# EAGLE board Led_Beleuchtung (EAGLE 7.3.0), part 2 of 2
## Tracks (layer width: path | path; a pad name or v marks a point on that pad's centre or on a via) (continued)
N$54  (via drill 0.35 pad 0.7) (continued)
  Bottom 0.7: v74.39,103.48 v75.04,102.83 v75.19,103.68 v74.54,104.33 v73.74,104.13 v74.39,103.48 | v74.39,103.48 74.64,103.73 | v64.14,114.98 v64.79,114.33 v64.94,115.18 v64.29,115.83 v63.49,115.63 v64.14,114.98 | v64.14,114.98 64.39,115.23
  Bottom 1.2: 74.64,103.73 74.64,105.03 64.44,115.23 64.39,115.23
N$55  (via drill 0.35 pad 0.7)
  Top 0.3: 70.54,99.66 v70.54,99.18 | 51.31,103.57 v50.96,103.57
  Top 0.7: v50.96,103.57 v50.96,102.65 v51.67,103.15 v51.67,104.06 v50.96,104.49 v50.96,103.57 | v50.96,103.57 51.32,103.57 | v69.69,99.33 v69.04,98.68 v69.89,98.53 v70.54,99.18 v70.34,99.98 v69.69,99.33 | v69.69,99.33 69.94,99.08
  Top 0.8: 71.54,100.64 D53.C
  Top 1.2: D53.C 70.54,99.66 | D54.A 51.31,103.57
  Bottom 0.3: 51.31,103.57 v50.96,103.57 | 70.08,99.18 v70.54,99.18
  Bottom 0.7: v50.96,103.57 v50.96,102.65 v51.67,103.15 v51.67,104.06 v50.96,104.49 v50.96,103.57 | v50.96,103.57 51.32,103.57 | v69.69,99.33 v69.04,98.68 v69.89,98.53 v70.54,99.18 v70.34,99.98 v69.69,99.33 | v69.69,99.33 69.94,99.08
  Bottom 1.2: 51.31,103.57 51.31,96.58 53.11,94.78 arc-33 62,93.25 64.87,93.97 70.08,99.18
N$56
  Top 0.7: IC16.3 53.94,119.88
  Top 0.8: 57.13,120.15 C67.2 56.53,120.33 53.94,119.88 | 57.87,117.15 R43.1
  Top 1.2: R43.1 57.13,120.15 | D54.C 51.31,110.76 52.57,112.02 54.36,112.02 57.87,115.52 57.87,117.15
N$57
  Top 0.5: IC17.1 15.22,88.5
  Top 0.8: 15.22,88.5 14.82,85.92 C69.1
  Top 1.2: C69.1 14.65,84.65 15.4,83.61 D56.C
N$58
  Top 1.2: D55.1 19.45,83.44 18.92,83.05 D56.A
N$59
  Top 0.78: IC17.6 12.08,89.18
  Top 0.8: 12.08,89.18 11.31,88.63 D57.C | 12.8,78.53 L27.1
  Top 1.2: D57.C C69.2 12.31,82.67 13.25,81.38 12.8,78.53
N$60
  Top 0.8: 4.22,87.05 C70.2 | 4.77,79.8 L27.2
  Top 1.2: 4.77,79.8 5.2,82.53 3.81,84.44 4.22,87.05 3.12,87.23 2.59,87.96 3.25,92.09 7.75,95.37 C71.1 16.14,97.34 16.61,97.81 16.79,97.98 30.69,97.98 D58.A
N$61
  Bottom 0.5: D6.A 27.63,15.54 R5.1
N$62  (via drill 0.35 pad 0.7)
  Top 0.6: IC17.3 15.59,90.73
  Top 0.7: v22.43,90.66 v22.43,91.58 v21.73,91.09 v21.73,90.17 v22.43,89.74 v22.43,90.66 | v22.43,90.66 22.08,90.66 | v23.35,74.29 v22.65,74.71 v22.65,75.63 v23.35,76.13 | v23.35,75.21 v23.35,76.13 | v23.35,74.29 v23.35,75.21 | v23.35,75.21 23,75.21 | 22.14,91.33 22.14,90.96 v22.43,90.66 | v23.35,76.13 24,76.13 24.09,76.03 | v23.35,74.29 24.19,74.28
  Top 0.8: 16.33,93.92 C71.2 16.04,93.48 15.59,90.73
  Top 1.2: 16.33,93.92 R45.1 19.93,93.49 22.14,91.33 | D59.C 24.54,75.21 v23.35,75.21
  Bottom 0.7: v22.43,90.66 v22.43,91.58 v21.73,91.09 v21.73,90.17 v22.43,89.74 v22.43,90.66 | v22.43,90.66 22.08,90.66 | v23.35,75.21 v23.35,76.13 v22.65,75.63 v22.65,74.71 v23.35,74.29 v23.35,75.21 | v23.35,75.21 23,75.21
  Bottom 1.2: 23,75.21 22.09,76.11 22.09,90.65 22.08,90.66
N$63
  Top 0.5: IC10.1 81.45,47.83
  Top 0.8: 81.45,47.83 83.29,49.66 C41.1
  Top 1.2: C41.1 84.17,50.59 84.17,51.87 D21.C
N$64
  Top 1.2: D20.1 81,54.39 81.66,54.39 D21.A
N$65
  Top 0.78: IC10.6 83.58,45.44
  Top 0.8: 83.58,45.44 84.71,45.41 86.06,46.76 D22.C | 89.27,54.45 L20.1
  Top 1.2: D22.C C41.2 87.14,50.73 87.14,52.32 89.27,54.45
N$66  (via drill 0.35 pad 0.7)
  Top 0.7: v70.54,45.99 v69.62,45.99 v70.12,45.28 v71.04,45.28 v71.46,45.99 v70.54,45.99 | v70.54,45.99 70.54,45.63 | v52.24,46.85 v51.81,46.14 v50.89,46.14 v50.4,46.85 | v51.32,46.85 v50.4,46.85 | v52.24,46.85 v51.32,46.85 | v51.32,46.85 51.32,46.49 | v50.4,46.85 50.4,47.78 50.59,47.78 | v52.24,46.85 52.24,47.73 51.84,47.73
  Top 0.8: 91.2,42.52 C42.2 | 95.04,48.71 L20.2
  Top 1.2: 95.04,48.71 92.98,46.65 92.98,44.3 91.2,42.52 91.99,41.73 91.99,40.83 89.02,37.87 83.46,37.87 C43.1 75.16,41.83 71.36,45.63 70.54,45.63 | D23.A 51.31,46.85 v51.32,46.85
  Bottom 0.7: v70.54,45.99 v69.62,45.99 v70.12,45.28 v71.04,45.28 v71.46,45.99 v70.54,45.99 | v70.54,45.99 70.54,45.63 | v51.32,46.85 v50.4,46.85 v50.89,46.14 v51.81,46.14 v52.24,46.85 v51.32,46.85 | v51.32,46.85 51.32,46.49
  Bottom 1.2: 51.32,46.49 52.23,45.58 70.49,45.58 70.54,45.63
N$67  (via drill 0.35 pad 0.7)
  Top 0.3: 51.31,54.86 v51.67,54.86
  Top 0.7: v69.34,58.83 v69.99,58.18 v70.14,59.03 v69.49,59.68 v68.69,59.48 v69.34,58.83 | v69.34,58.83 69.59,59.08 | v50.96,54.37 v50.96,53.45 v51.67,53.95 v51.67,54.86 v50.96,55.29 v50.96,54.37 | v50.96,54.37 51.32,54.37
  Top 0.8: D23.C
  Top 1.2: 69.59,59.08 D24.A | D23.C 51.31,54.86
  Route3 0.3: 51.3,54.37 v50.96,54.37
  Route3 0.7: v69.34,58.83 v69.99,58.18 v70.14,59.03 v69.49,59.68 v68.69,59.48 v69.34,58.83 | v69.34,58.83 69.59,59.08 | v50.96,54.37 v50.96,53.45 v51.67,53.95 v51.67,54.86 v50.96,55.29 v50.96,54.37 | v50.96,54.37 51.32,54.37
  Route3 1.2: 69.59,59.08 66.31,62.36 63.61,63.08 arc-35 53.11,61.01 51.3,59.21 51.3,54.37
N$68
  Top 0.7: IC10.3 79.84,46.23
  Top 0.8: 77.37,44.08 C43.2 77.99,44.28 79.84,46.23 | 75.43,46.05 R31.1
  Top 1.2: R31.1 77.37,44.08 | D24.C 75.47,53.2 75.47,51.76 73.4,49.7 73.4,48.08 75.43,46.05
N$69
  Top 0.8: 26.42,108.22 C45.1 26.42,108.22 | IC11.1 26.42,108.22
  Top 1.2: C45.1 25.54,107.28 25.54,106 D26.C
N$70
  Top 1.2: D25.1 28.71,103.49 28.05,103.49 D26.A
N$71
  Top 0.78: IC11.6 26.31,112.33
  Top 0.8: D27.C 25.04,112.33 26.31,112.33 | 20.44,103.43 L21.1
  Top 1.2: D27.C C45.2 22.66,107.24 22.66,105.65 20.44,103.43
N$72  (via drill 0.35 pad 0.7)
  Top 0.7: v57.7,110.89 v58.12,111.59 v59.04,111.59 v59.54,110.89 | v58.62,110.89 v59.54,110.89 | v57.7,110.89 v58.62,110.89 | v58.62,110.89 58.62,111.24 | v40.99,111.82 v41.91,111.82 v41.42,112.52 v40.5,112.52 v40.07,111.82 v40.99,111.82 | v40.99,111.82 40.99,112.17 | v57.7,110.89 57.7,110.03 57.69,110.03 | v59.54,110.89 59.54,109.78 59.39,109.78
  Top 0.8: 18.52,115.36 C46.2 | 14.7,109.17 L21.2
  Top 1.2: 18.52,115.36 17.72,116.15 17.72,117.05 20.69,120.01 26.26,120.01 C47.1 34,116.05 37.87,112.17 40.99,112.17 | C46.2 16.74,113.55 16.74,111.21 14.7,109.17 | D28.A 58.67,110.89 v58.62,110.89
  Bottom 0.7: v58.62,110.89 v59.54,110.89 v59.04,111.59 v58.12,111.59 v57.7,110.89 v58.62,110.89 | v58.62,110.89 58.62,111.24 | v40.99,111.82 v41.91,111.82 v41.42,112.52 v40.5,112.52 v40.07,111.82 v40.99,111.82 | v40.99,111.82 40.99,112.17
  Bottom 1.2: 58.62,111.24 57.67,112.18 41.01,112.18 40.99,112.17
N$73  (via drill 0.35 pad 0.7)
  Top 0.3: 40.16,98.93 v40.64,98.93 | 58.67,103.4 v59.02,103.4
  Top 0.7: v59.02,103.4 v59.02,104.32 v58.31,103.82 v58.31,102.9 v59.02,102.48 v59.02,103.4 | v59.02,103.4 58.67,103.4 | v40.64,98.93 v39.99,99.58 v39.84,98.73 v40.49,98.08 v41.29,98.28 v40.64,98.93 | v40.64,98.93 40.39,98.68
  Top 0.8: D28.C
  Top 1.2: D29.A 40.16,98.93 | D28.C 58.67,103.4
  Route3 0.3: 58.67,103.4 v59.02,103.4 | 40.64,98.44 v40.64,98.93
  Route3 0.7: v59.02,103.4 v59.02,104.32 v58.31,103.82 v58.31,102.9 v59.02,102.48 v59.02,103.4 | v59.02,103.4 58.67,103.4 | v40.64,98.93 v39.99,99.58 v39.84,98.73 v40.49,98.08 v41.29,98.28 v40.64,98.93 | v40.64,98.93 40.39,98.68
  Route3 1.2: 58.67,103.4 58.67,98.55 56.88,96.76 arc33 46.73,94.87 43.68,95.41 40.64,98.44
N$74
  Top 0.7: IC11.3 29.89,111.68
  Top 0.8: 32.35,113.8 C47.2 32.13,113.92 29.89,111.68 | 34.28,111.81 R33.1
  Top 1.2: R33.1 32.35,113.8 | D29.C 34.25,104.85 34.25,106.81 35.77,108.34 35.77,110.32 34.28,111.81
N$75
  Top 0.5: IC12.1 92.36,94.53
  Top 0.8: 92.36,94.53 91.2,96.8 C49.1
  Top 1.2: C49.1 90.59,97.94 89.37,98.33 D31.C
N$76
  Top 1.2: D30.1 86,96.09 86.21,96.72 D31.A
N$77
  Top 0.78: IC12.6 95.29,95.77
  Top 0.8: 88.5,103.97 L22.1 | 95.29,95.77 95.63,96.67 94.66,98.59 D32.C
  Top 1.2: D32.C C49.2 91.49,100.57 89.98,101.06 88.5,103.97
N$78
  Top 0.8: 95.74,107.66 L22.2 | 100.44,102.12 C50.2
  Top 1.2: C50.2 99.33,104.26 97.11,104.98 95.74,107.66 | 100.44,102.12 101.44,102.63 102.29,102.35 104.2,98.61 102.48,93.32 C51.1 97.48,86.9 D33.A
N$79  (via drill 0.35 pad 0.7)
  Top 0.3: 79.7,75.2 v79.36,74.86 | 74.8,93.48 v74.29,93.48
  Top 0.7: v75.14,93.33 v75.79,93.98 v74.94,94.13 v74.29,93.48 v74.49,92.68 v75.14,93.33 | v75.14,93.33 74.89,93.58 | v79.36,74.86 v80.28,74.86 v79.78,75.56 v78.86,75.56 v78.44,74.86 v79.36,74.86 | v79.36,74.86 79.36,75.21
  Top 0.8: D34.A | D33.C
  Top 1.2: D33.C 79.7,75.2 | D34.A 74.8,93.48
  Route3 0.3: 74.65,93.33 v75.14,93.33 | 79.78,75.2 v79.78,75.56
  Route3 0.7: v75.14,93.33 v75.79,93.98 v74.94,94.13 v74.29,93.48 v74.49,92.68 v75.14,93.33 | v75.14,93.33 74.89,93.58 | v79.36,74.86 v80.28,74.86 v79.78,75.56 v78.86,75.56 v78.44,74.86 v79.36,74.86 | v79.36,74.86 79.36,75.21
  Route3 1.2: 74.65,93.33 71.52,90.2 70.8,87.51 arc-35 72.86,77 74.66,75.2 79.78,75.2
N$80
  Top 0.7: IC12.3 93.44,92.38
  Top 0.8: 92.37,88.17 R35.1 | 93.44,92.38 94.75,89.98 C51.2
  Top 1.2: 92.37,88.17 C51.2 | D34.C 80.28,98.97 82.31,98.97 88.04,87.69 89.93,87.06 R35.1
N$81
  Top 0.5: IC13.1 17.78,63.57
  Top 0.8: 17.78,63.57 18.95,61.25 C53.1
  Top 1.2: C53.1 19.56,60.12 20.78,59.73 D36.C
N$82
  Top 1.2: D35.1 24.15,61.97 23.95,61.34 D36.A
N$83
  Top 0.78: IC13.6 14.86,62.29
  Top 0.8: 21.66,54.09 L23.1 | 14.86,62.29 14.52,61.38 D37.C
  Top 1.2: D37.C C53.2 18.66,57.49 20.18,57 21.66,54.09
N$84
  Top 0.8: 14.42,50.4 L23.2 | 9.71,55.94 C54.2
  Top 1.2: C54.2 10.77,53.91 12.99,53.19 14.42,50.4 | 9.71,55.94 8.72,55.43 7.86,55.71 5.96,59.44 7.68,64.74 C55.1 12.68,71.06 D38.A
N$85  (via drill 0.35 pad 0.7)
  Top 0.3: 30.63,82.58 v30.63,82.91 | 34.5,63.78 v35.14,63.78
  Top 0.7: v34.94,64.58 v34.29,63.93 v35.14,63.78 v35.79,64.43 v35.59,65.23 v34.94,64.58 | v34.94,64.58 35.19,64.33 | v30.63,82.91 v29.71,82.91 v30.2,82.21 v31.12,82.21 v31.55,82.91 v30.63,82.91 | v30.63,82.91 30.63,82.56
  Top 0.8: D39.A 33.52,62.64 33.44,62.72 | D38.C 28.26,82.57
  Top 1.2: D38.C 30.63,82.58 | 33.44,62.72 34.5,63.78
  Route3 0.3: 35.48,64.58 v34.94,64.58 | 30.96,82.58 v30.63,82.91
  Route3 0.7: v34.94,64.58 v34.29,63.93 v35.14,63.78 v35.79,64.43 v35.59,65.23 v34.94,64.58 | v34.94,64.58 35.19,64.33 | v30.63,82.91 v29.71,82.91 v30.2,82.21 v31.12,82.21 v31.55,82.91 v30.63,82.91 | v30.63,82.91 30.63,82.56
  Route3 1.2: 35.48,64.58 38.47,67.57 39.19,70.26 arc-35 37.12,80.77 35.31,82.58 30.96,82.58
N$86
  Bottom 1.4: 26.99,27.93 31.71,27.93 D1.A1 D1.A2 34.21,27.52 34.21,27.19 33.35,26.34 27.95,26.34 PJ1.1.2 32.8,27.14 33.19,27.53
  Bottom 3: PJ1.1.1 PJ1.1.2
N$87
  Top 0.7: IC13.3 16.69,65.68
  Top 0.8: 17.79,69.89 R37.1 | 16.69,65.68 15.39,68.08 C55.2
  Top 1.2: C55.2 17.79,69.89 | R37.1 19.97,70.8 21.95,70.08 27.67,58.8 29.68,58.8 D39.C
N$88
  Bottom 0.5: D7.A 30.27,15.51 R6.1
N$89
  cutout Bottom: 56.28,37.55 58.63,40.79 arc-180 60.3,39.56 57.95,36.32 arc-180
  cutout Bottom: 31.88,44.59 35.69,45.83 arc-180 36.33,43.85 32.52,42.62 arc-180
  cutout Bottom: 16.33,65.03 20.13,63.8 arc-180 19.51,61.82 15.71,63.06 arc-180
  cutout Bottom: 14.89,90.47 17.24,87.24 arc-180 15.6,86.04 13.25,89.27 arc-180
  cutout Bottom: 29.25,112.12 29.46,108.12 arc-180 27.39,107.87 27.23,111.92 arc-180
  cutout Bottom: 53.46,120.5 51.11,117.26 arc-180 49.41,118.44 51.77,121.68 arc-180
  cutout Bottom: 78.26,113.56 74.46,112.32 arc-180 73.81,114.28 77.62,115.51 arc-180
  cutout Bottom: 93.84,93.04 90.04,94.27 arc-180 90.68,96.23 94.48,94.99 arc-180
  cutout Bottom: 94.89,67.12 92.54,70.35 arc-180 94.21,71.56 96.56,68.32 arc-180
N$90
  Bottom 0.5: D8.A 32.5,15.56 R7.1
N$91
  Top 0.5: OC1.3 81.32,29.77 80.04,28.48 80.04,23.67 R23.1
N$92
  Top 0.3: U1.1 67,21.46 JP1.2
N$93
  Top 0.3: R24.2 77.09,18.54
  Top 0.5: OC2.3 77.07,14.2 R24.2
N$94
  Top 0.3: U1.2 55.13,20.59 55.54,20.18 66.74,20.18 69.84,23.28 70.94,23.28 71.69,24.03 71.69,25.94 JP1.4
N$95
  Top 0.3: IC5.30 80.12,21.89 R23.2
N$97  (via drill 0.35 pad 0.7)
  Top 0.3: IC5.2 83.35,19.73 v83.74,19.33 | R22.2 81.95,10.99
  Top 0.5: 81.95,10.99 OC2.4 | v84.24,11.58 83.6,10.94 R22.2
  Bottom 0.5: v83.74,19.33 84.24,18.83 v84.24,11.58
N$98  (via drill 0.35 pad 0.7)
  Top 0.3: R30.2 v81.66,41.64 81.66,42.53 82.06,42.93 IC10.4
  Route3 0.3: v81.66,41.64 79.24,39.19 79.22,39.19 JP9.2
N$99  (via drill 0.35 pad 0.7)
  Top 0.3: R32.2 v28.05,116.24 28.05,115.34 27.69,114.98 27.69,113.63 IC11.4
  Route3 0.3: v28.05,116.24 30.3,118.49 JP10.2
N$100  (via drill 0.35 pad 0.7)
  Top 0.3: R34.2 v98.33,92.78 97.48,93.05 97.24,93.53 IC12.4
  Route3 0.3: v98.33,92.78 99.95,89.72 JP11.2
N$101  (via drill 0.35 pad 0.7)
  Top 0.3: 14.31,64.27 IC13.4 12.98,64.41 12.68,65 v11.82,65.28 R36.2
  Route3 0.3: v11.82,65.28 10.15,68.56 JP12.2
N$102  (via drill 0.35 pad 0.7)
  Top 0.3: R38.2 v54.71,33.4 55.24,34.13 55.77,34.21 IC14.4
  Route3 0.3: v54.71,33.4 51.34,32.87 JP13.2
N$103  (via drill 0.35 pad 0.7)
  Top 0.3: R40.2 v98.31,64.38 97.78,65.11 97.87,65.65 IC15.4
  Route3 0.3: v98.31,64.38 97.77,61 JP14.2
N$104  (via drill 0.35 pad 0.7)
  Top 0.3: R42.2 v55.09,124.65 54.56,123.92 54.09,123.83 IC16.4
  Route3 0.3: v55.09,124.65 58,125.12 JP15.2
N$105  (via drill 0.35 pad 0.7)
  Top 0.3: R44.2 v11.42,93.37 11.95,92.64 11.86,92.06 IC17.4
  Route3 0.3: v11.42,93.37 11.92,96.54 JP16.2
N$106  (via drill 0.35 pad 0.7)
  Top 0.3: R46.2 v82.09,116.03 81.24,115.75 80.74,115.98 IC18.4
  Route3 0.3: v82.09,116.03 84.94,114.57 JP18.2
N$107  (via drill 0.35 pad 0.7)
  Top 0.3: R48.2 v28.02,42.14 28.88,42.41 29.39,42.15 IC19.4
  Route3 0.3: v28.02,42.14 24.97,43.69 JP17.2
N$108
  cutout Bottom: 80.55,46.01 80.55,50.01 arc-180 82.55,50.01 82.55,46.01 arc-180
N$112
  cutout Route2: 48.04,19.51 48.12,19.51 arc90 48.92,20.31 48.92,20.33 arc90 48.12,21.13 48.04,21.13 arc90 47.19,20.28 47.19,20.26 arc90 47.94,19.51
N$113
  cutout Route3: 49.72,19.56 arc-90 49.07,20.21 49.07,20.28 arc-90 49.74,20.96 49.77,20.96 49.79,20.96 arc-90 50.44,20.31 50.44,20.28 arc-90
N$117
  cutout Route3: 37.54,26.63 37.54,26.03 65.64,26.03 67.69,28.08 78.19,28.08 78.19,28.68 67.39,28.68 65.34,26.63
N$118
  pour Bottom (rank 2, no thermals): 54.97,41.38 54.34,41.38 54.34,26.38 54.94,26.38 54.97,26.38
NMI  (via drill 0.35 pad 0.7)
  Top 0.3: U1.26 42.52,15.05 v41.99,15.58 | 35.23,16.73 R9.2 36.46,16.7 v36.49,16.73
  Bottom 0.3: v41.99,15.58 40.84,16.73 v36.49,16.73
PTA5
  Top 0.3: JP5.4 41.32,14.57 U1.27
PTA12
  Top 0.3: JP5.6 41.53,14.06 U1.28
PTA13
  Top 0.3: JP5.5 39.07,11.73 41.09,11.73 42.91,13.56 U1.29
PTB0
  Top 0.3: U1.35 49.14,5.63 48.04,4.53 48.04,2.69 JP8.8
PTB1
  Top 0.3: U1.36 49.62,4.27 JP8.7
PTB2
  Top 0.3: U1.37 50.13,5 50.59,4.53 50.59,2.68 JP8.6
PTB3
  Top 0.3: U1.38 50.64,5.18 JP8.5
PTB16
  Top 0.3: U1.39 51.12,6.46 53.09,4.48 53.09,2.72 JP8.4
PTC0
  Top 0.3: U1.43 53.13,7.6 54.54,6.18 56.69,6.18 58.29,4.58 58.29,2.95 JP7.8
PTC1
  Top 0.3: U1.44 53.63,7.89 54.79,6.73 57.05,6.73 JP7.7
PTC2
  Top 0.3: U1.45 54.14,8.18 55.04,7.28 58.34,7.28 61.09,4.53 61.09,2.69 JP7.6
PTC3
  Top 0.3: U1.46 54.62,8.45 55.29,7.78 58.54,7.78 JP7.5
PTC4
  Top 0.3: JP7.4 63.59,2.73 63.59,4.48 57.52,10.56 U1.49
PTC5
  Top 0.3: U1.50 58.41,12.57 59.04,11.93 59.04,9.82 JP7.3
PTC6
  Top 0.3: U1.51 58.65,13.07 59.74,11.98 59.74,9.88 64.44,5.18 65.49,5.18 66.09,4.58 66.09,2.77 JP7.2
PTC7
  Top 0.3: U1.52 58.92,13.56 60.49,11.98 60.49,10.03 64.74,5.78 65.62,5.78 JP7.1
PTD0
  Top 0.3: JP6.6 71.62,15.63 67.14,15.63 66.04,14.53 63.34,14.53 61.81,16.07 U1.57
PTD1
  Top 0.3: U1.58 62.15,16.58 63.64,15.08 65.79,15.08 67.61,16.9 JP6.5
PTD4
  Top 0.3: U1.61 71.52,18.08 JP6.4
PTD5
  Top 0.3: U1.62 69.47,18.56 JP6.3
PTD6
  Top 0.3: U1.63 68.13,19.07 69.74,20.68 71.59,20.68 JP6.2
PTD7
  Top 0.3: U1.64 67.38,19.58 69.79,21.98 JP6.1
PTE23
  Top 0.3: U1.12 JP4.4 | JP4.4
PTE24
  Top 0.3: U1.20 40.47,18.08 JP5.2
PTE25
  Top 0.3: U1.21 41.88,17.57 41.04,16.73 39.15,16.73 JP5.1
PTE29
  Top 0.3: JP4.6 47.59,23.58 46.84,22.83 46.84,20.68 46.24,20.08 U1.17 | U1.17
PTE30
  Top 0.3: U1.18 47.03,19.07 47.34,19.38 47.34,22.43 48.89,23.98 48.89,25.98 JP4.3
PTE31
  Top 0.3: U1.19 45.42,18.56 45.14,18.83 45.14,19.83 46.34,21.03 46.34,25.97 JP4.5
PWM_IR  (via drill 0.35 pad 0.7)
  Top 0.3: U1.11 50.64,23.23 51.39,23.98 51.39,27.88 49.94,29.33 v47.64,29.33
  Route3 0.3: JP17.1 22.04,42.43 24.54,41.08 26.14,36.18 39.74,29.08 v47.64,29.33 44.84,33.43 42.74,44.98 46.74,54.68 51.94,63.93 53.54,66.48 58.34,67.18 63.24,69.98 65.74,73.13 67.39,79.03 v66.24,83.73 | JP18.1 85.04,102.78 88.54,95.73 v89.24,93.28
  Bottom 0.3: v89.24,93.28 v66.24,83.73
PWM_UV  (via drill 0.35 pad 0.7)
  Top 0.3: U1.9 51.63,22.32 52.34,23.03 53.44,23.03 54.59,24.18 54.59,25.18 v55.74,26.33
  Route3 0.3: v55.74,26.33 57.29,27.88 64.59,27.88 JP9.1 73.84,50.18 84.54,61.83 89.39,77.63 JP11.1 88.14,87.68 80.39,103.38 62.14,112.48 44.99,113.18 JP10.1 35.89,108.48 25.14,94.88 21.79,82.53 JP12.1
PWM_WHITE  (via drill 0.35 pad 0.7)
  Top 0.3: U1.10 51.12,22.56 52.09,23.53 53.19,23.53 54.09,24.43 54.09,27.63 52.99,28.73 51.63,28.73 JP13.1 | v75.29,32.93 v68.84,34.48
  Route3 0.3: JP16.1 8.94,104.48 13.89,111.28 27.44,123.63 38.34,128.48 51.69,130.33 JP15.1 69.29,129.73 84.07,121.53 88.97,116.41 93.82,111.63 98.39,106.66 103.59,96.33 107.14,79.78 104.99,66.23 JP14.1 97.94,49.08 87.84,39.18 v75.29,32.93 | v68.84,34.48 49.74,30.63 JP13.1
SWD_CLK_TGTMCU  (via drill 0.35 pad 0.7)
  Top 0.3: U1.22 44.87,17.06 v44.54,16.73 | PROG.4 37.7,22.74 37.34,22.38 37.34,20.73 38.19,19.88 43.79,19.88 v44.14,19.53
  Bottom 0.3: v44.54,16.73 44.14,17.13 v44.14,19.53
SWD_DIO_TGTMCU  (via drill 0.35 pad 0.7)
  Top 0.3: U1.25 43.26,15.56 v42.49,16.33 | 39.49,21.46 PROG.2 39.51,20.87 39.79,20.58 v42.49,20.58
  Bottom 0.3: 42.44,16.38 v42.49,16.33 v42.49,20.58
SWD_RST_TGTMCU  (via drill 0.35 pad 0.7)
  Top 0.3: v48.99,11.83 48.63,11.47 U1.34 | PROG.10 39.49,26.57 39.49,27.03 40.09,27.63 44.64,27.63 v45.59,26.68
  Bottom 0.3: v48.99,11.83 48.99,13.48 | 48.99,13.48 48.99,25.28 48.34,25.93 46.34,25.93 v45.59,26.68 | R17.2 48.04,13.48 48.99,13.48 | C13.2 50.09,13.48 48.99,13.48
TH_D23  (via drill 0.35 pad 0.7)
  Top 0.7: D23.TH 51.49,49.94 v51.49,49.81 | v54.09,52.78 54.09,47.53 v53.67,47.53 53.67,52.78 v54.09,52.78 | v48.94,52.81 48.94,47.46 v48.52,47.46 48.52,52.81 v48.94,52.81
  other vias: 48.97,50.43 49.32,49.81 49.69,50.43 50.04,49.81 50.42,50.43 50.77,49.81 51.14,50.43 51.87,50.43 52.22,49.81 52.59,50.43 52.94,49.81 53.32,50.43 53.67,49.81 54.04,50.43 54.09,49.23 53.64,48.66 54.09,48.11 53.67,51.06 54.09,51.63 53.67,52.21 48.59,49.81 48.94,49.18 48.52,48.61 48.94,48.03 48.54,51.01 48.94,51.61 48.54,52.21
  pour Bottom (no thermals): 54.77,41.73 54.77,53.18 44.62,53.18 41.02,44.46 43.49,43.56 46.49,42.71 50.67,41.98
TH_D24  (via drill 0.35 pad 0.7)
  Top 0.3: v72.39,56.06 D24.TH
  Top 0.7: v72.82,59.8 76.53,56.09 v76.23,55.79 72.52,59.5 v72.82,59.8 | v69.16,56.18 72.94,52.4 v72.64,52.1 68.86,55.88 v69.16,56.18
  other vias: 70.85,54.52 71.54,54.32 71.37,55.03 72.06,54.84 71.88,55.54 72.57,55.35 73.08,55.86 72.9,56.57 73.59,56.37 73.42,57.08 74.11,56.89 73.93,57.59 74.62,57.4 74.44,58.11 75.33,57.29 75.41,56.57 76.12,56.5 73.73,58.28 73.63,58.99 72.92,59.1 71.03,53.81 71.72,53.62 71.83,52.91 72.53,52.8 70.15,54.62 70.01,55.33 69.3,55.47
  pour Bottom (no thermals): 81.09,52.48 72.99,60.58 65.81,53.4 69.44,44.69 71.82,45.8 74.55,47.32 78.01,49.76
TH_D28  (via drill 0.35 pad 0.7)
  Top 0.3: D28.TH v58.52,107.96
  Top 0.7: v61.47,110.31 61.47,105.06 v61.04,105.06 61.04,110.31 v61.47,110.31 | v56.32,110.33 56.32,104.98 v55.89,104.98 55.89,110.33 v56.32,110.33
  other vias: 56.34,107.96 56.69,107.33 57.07,107.96 57.42,107.33 57.79,107.96 58.14,107.33 58.87,107.33 59.24,107.96 59.59,107.33 59.97,107.96 60.32,107.33 60.69,107.96 61.04,107.33 61.42,107.96 61.47,106.76 61.02,106.18 61.47,105.63 61.04,108.58 61.47,109.16 61.04,109.73 55.97,107.33 56.32,106.71 55.89,106.13 56.32,105.56 55.92,108.53 56.32,109.13 55.92,109.73
  pour Bottom (no thermals): 55.22,116.01 55.22,104.56 65.37,104.56 68.97,113.28 66.49,114.18 63.49,115.03 59.32,115.76
TH_D29  (via drill 0.35 pad 0.7)
  Top 0.3: v37.61,101.78 D29.TH
  Top 0.7: v37.34,105.72 41.05,102.01 v40.75,101.71 37.04,105.42 v37.34,105.72 | v33.68,102.09 37.47,98.31 v37.16,98.01 33.38,101.79 v33.68,102.09
  other vias: 35.38,100.43 36.07,100.24 35.89,100.95 36.58,100.75 36.4,101.46 37.09,101.26 36.92,101.97 37.43,102.48 38.12,102.29 37.94,103 38.63,102.8 38.45,103.51 39.14,103.31 38.97,104.02 39.85,103.21 39.94,102.48 40.65,102.41 38.26,104.2 38.15,104.91 37.45,105.01 35.56,99.73 36.25,99.53 36.35,98.82 37.06,98.72 34.67,100.54 34.53,101.25 33.82,101.39
  pour Bottom (no thermals): 28.9,105.29 36.99,97.19 44.17,104.37 40.55,113.08 38.16,111.97 35.44,110.45 31.97,108.01
TH_D33  (via drill 0.35 pad 0.7)
  Top 0.3: v84.04,75.38 D33.TH
  Top 0.7: v81.07,77.98 86.32,77.98 v86.32,77.56 81.07,77.56 v81.07,77.98 | v81.04,72.83 86.39,72.83 v86.39,72.41 81.04,72.41 v81.04,72.83
  other vias: 83.42,72.86 84.04,73.21 83.42,73.58 84.04,73.93 83.42,74.31 84.04,74.66 83.42,75.03 83.42,75.76 84.04,76.11 83.42,76.48 84.04,76.83 83.42,77.21 84.04,77.56 83.42,77.93 84.62,77.98 85.19,77.53 85.74,77.98 82.79,77.56 82.22,77.98 81.64,77.56 84.04,72.48 84.67,72.83 85.24,72.41 85.82,72.83 82.84,72.43 82.24,72.83 81.64,72.43
  pour Bottom (no thermals): 92.12,78.66 80.67,78.66 80.67,68.51 89.39,64.91 90.29,67.38 91.14,70.38 91.87,74.56
TH_D34  (via drill 0.35 pad 0.7)
  Top 0.3: D34.TH v77.81,96.29
  Top 0.7: v74.06,96.72 77.78,100.43 v78.08,100.13 74.36,96.42 v74.06,96.72 | v77.69,93.06 81.47,96.84 v81.77,96.54 77.99,92.76 v77.69,93.06
  other vias: 79.35,94.76 79.54,95.44 78.84,95.27 79.03,95.96 78.32,95.78 78.52,96.47 78.01,96.98 77.3,96.81 77.49,97.5 76.79,97.32 76.98,98.01 76.27,97.83 76.47,98.52 75.76,98.34 76.57,99.23 77.3,99.32 77.37,100.02 75.58,97.64 74.88,97.53 74.77,96.82 80.06,94.93 80.25,95.62 80.96,95.73 81.06,96.43 79.24,94.05 78.54,93.91 78.4,93.2
  pour Bottom (no thermals): 81.39,104.98 73.3,96.88 80.48,89.71 89.19,93.33 88.08,95.72 86.56,98.44 84.12,101.9
TH_D38  (via drill 0.35 pad 0.7)
  Top 0.3: v25.92,82.41 D38.TH
  Top 0.7: v23.57,85.36 28.82,85.36 v28.82,84.93 23.57,84.93 v23.57,85.36 | v23.54,80.21 28.89,80.21 v28.89,79.78 23.54,79.78 v23.54,80.21
  other vias: 25.92,80.23 26.54,80.58 25.92,80.96 26.54,81.31 25.92,81.68 26.54,82.03 26.54,82.76 25.92,83.13 26.54,83.48 25.92,83.86 26.54,84.21 25.92,84.58 26.54,84.93 25.92,85.31 27.12,85.36 27.69,84.91 28.24,85.36 25.29,84.93 24.72,85.36 24.14,84.93 26.54,79.86 27.17,80.21 27.74,79.78 28.32,80.21 25.34,79.81 24.74,80.21 24.14,79.81
  pour Bottom (no thermals): 17.84,79.11 29.29,79.11 29.29,89.26 20.57,92.86 19.67,90.38 18.82,87.38 18.09,83.21
TH_D39  (via drill 0.35 pad 0.7)
  Top 0.3: v31.93,60.83 D39.TH
  Top 0.7: v28.18,61.25 31.89,64.96 v32.19,64.66 28.48,60.95 v28.18,61.25 | v31.8,57.59 35.59,61.37 v35.89,61.07 32.11,57.29 v31.8,57.59
  other vias: 33.47,59.29 33.66,59.98 32.95,59.8 33.15,60.49 32.44,60.31 32.64,61 32.12,61.52 31.42,61.34 31.61,62.03 30.9,61.85 31.1,62.54 30.39,62.37 30.58,63.05 29.88,62.88 30.69,63.76 31.42,63.85 31.49,64.56 29.7,62.17 28.99,62.06 28.89,61.36 34.17,59.47 34.37,60.16 35.07,60.26 35.18,60.97 33.36,58.58 32.65,58.44 32.51,57.73
  pour Bottom (no thermals): 28.56,52.79 36.66,60.89 29.48,68.06 20.77,64.44 21.88,62.05 23.4,59.33 25.84,55.87
TH_D43  (via drill 0.35 pad 0.7)
  Top 0.3: v37.3,56.29 D43.TH
  Top 0.7: v40.2,56.08 37.12,53 v37.39,52.74 40.47,55.81 v40.2,56.08 | v37.12,59.15 34.05,56.08 v34.31,55.81 37.39,58.89 v37.12,59.15
  other vias: 35.39,57.38 39.1,54.49 38.5,55.09 37.9,55.69 36.7,56.89 36.22,58.22 36.1,57.49 35.99,56.78 35.2,56.7 36.59,56.18 37.2,55.58 37.8,54.98 38.4,54.38 34.49,56.52 36.93,58.43 38.29,53.67 39.32,55.19 40.02,55.37 37.58,53.46
  pour Bottom (no thermals): 28.88,52.47 36.98,60.57 44.16,53.39 40.53,44.68 38.15,45.79 35.42,47.31 31.96,49.75
TH_D44  (via drill 0.35 pad 0.7)
  Top 0.3: D44.TH 58.68,49.83 v58.89,49.83
  Top 0.7: v60.67,52.31 60.67,47.96 v61.04,47.96 61.04,52.31 v60.67,52.31 | v56.32,52.31 56.32,47.96 v56.69,47.96 56.69,52.31 v56.32,52.31
  other vias: 56.34,49.83 61.02,50.41 60.17,50.41 59.32,50.41 58.47,50.41 57.62,50.41 56.34,51.01 56.77,50.41 57.19,49.83 56.69,49.21 58.04,49.83 59.74,49.83 60.59,49.83 56.32,48.58 56.69,51.66 61.02,49.26 60.67,51.06 61.04,51.68 60.67,48.61
  pour Bottom (no thermals): 55.22,41.73 55.22,53.18 65.37,53.18 68.97,44.46 66.49,43.56 63.49,42.71 59.32,41.98
TH_D48  (via drill 0.35 pad 0.7)
  Top 0.3: v78.28,61.1 D48.TH
  Top 0.7: v78.07,58.2 74.99,61.27 v74.73,61.01 77.8,57.93 v78.07,58.2 | v81.14,61.27 78.07,64.35 v77.8,64.08 80.88,61.01 v81.14,61.27
  other vias: 79.38,63.01 76.48,59.29 77.08,59.9 77.68,60.5 78.88,61.7 80.21,62.18 79.48,62.3 78.78,62.41 78.69,63.2 78.17,61.8 77.57,61.2 76.97,60.6 76.37,60 78.51,63.91 80.42,61.47 75.66,60.11 77.18,59.08 77.36,58.38 75.45,60.81
  pour Bottom (no thermals): 81.41,52.8 73.31,60.9 80.49,68.07 89.2,64.45 88.09,62.06 86.57,59.34 84.13,55.88
TH_D49  (via drill 0.35 pad 0.7)
  Top 0.3: v84.04,82.78 D49.TH
  Top 0.7: v85.94,80.58 81.59,80.58 v81.59,80.21 85.94,80.21 v85.94,80.58 | v85.94,84.93 81.59,84.93 v81.59,84.56 85.94,84.56 v85.94,84.93
  other vias: 83.47,84.91 84.04,80.23 84.04,81.08 84.04,81.93 84.04,83.63 84.64,84.91 84.04,84.48 83.47,84.06 82.84,84.56 83.47,83.21 83.47,82.36 83.47,81.51 83.47,80.66 82.22,84.93 85.29,84.56 82.89,80.23 84.69,80.58 85.32,80.21 82.24,80.58
  pour Bottom (no thermals): 92.12,79.11 80.67,79.11 80.67,89.26 89.39,92.86 90.29,90.38 91.14,87.38 91.87,83.21
TH_D53  (via drill 0.35 pad 0.7)
  Top 0.3: D53.TH v72.66,101.49
  Top 0.7: v75.67,101.98 72.59,98.91 v72.86,98.64 75.93,101.72 v75.67,101.98 | v72.59,105.06 69.51,101.98 v69.78,101.72 72.86,104.79 v72.59,105.06
  other vias: 70.86,103.29 74.57,100.39 73.97,100.99 73.37,101.59 72.77,102.2 72.17,102.8 71.69,104.12 71.57,103.4 71.46,102.69 70.66,102.6 72.06,102.09 73.26,100.89 73.86,100.29 69.96,102.43 72.4,104.33 73.76,99.58 74.78,101.1 75.49,101.28 73.05,99.37
  pour Bottom (no thermals): 81.08,105.3 72.98,97.2 65.8,104.38 69.43,113.09 71.81,111.98 74.54,110.46 78,108.02
TH_D54  (via drill 0.35 pad 0.7)
  Top 0.3: D54.TH v51.52,107.36
  Top 0.7: v49.32,105.46 49.32,109.81 v48.94,109.81 48.94,105.46 v49.32,105.46 | v53.67,105.46 53.67,109.81 v53.29,109.81 53.29,105.46 v53.67,105.46
  other vias: 53.64,107.93 48.97,107.36 49.82,107.36 50.67,107.36 52.37,107.36 53.64,106.76 53.22,107.36 52.79,107.93 53.29,108.56 51.94,107.93 51.09,107.93 50.24,107.93 49.39,107.93 53.67,109.18 53.29,106.11 48.97,108.51 49.32,106.71 48.94,106.08 49.32,109.16
  pour Bottom (no thermals): 54.77,116.01 54.77,104.56 44.62,104.56 41.02,113.28 43.49,114.18 46.49,115.03 50.67,115.76
TH_D58  (via drill 0.35 pad 0.7)
  Top 0.3: v31.7,96.68 D58.TH
  Top 0.7: v32.19,93.68 29.12,96.76 v28.85,96.49 31.93,93.41 v32.19,93.68 | v35.27,96.76 32.19,99.83 v31.93,99.57 35,96.49 v35.27,96.76
  other vias: 33.5,98.49 30.6,94.78 31.2,95.38 31.8,95.98 32.4,96.58 33,97.18 34.33,97.66 33.61,97.78 32.9,97.89 32.81,98.68 32.3,97.29 31.1,96.08 30.49,95.48 32.63,99.39 34.54,96.95 29.79,95.59 31.31,94.56 31.48,93.86 29.58,96.3
  pour Bottom (no thermals): 28.58,104.97 36.68,96.87 29.5,89.7 20.78,93.32 21.9,95.71 23.42,98.43 25.86,101.89
TH_D59  (via drill 0.35 pad 0.7)
  Top 0.3: v25.94,74.98 D59.TH
  Top 0.7: v28.42,73.21 24.07,73.21 v24.07,72.83 28.42,72.83 v28.42,73.21 | v28.42,77.56 24.07,77.56 v24.07,77.18 28.42,77.18 v28.42,77.56
  other vias: 25.94,77.53 26.52,72.86 26.52,73.71 26.52,74.56 26.52,75.41 26.52,76.26 27.12,77.53 26.52,77.11 25.94,76.68 25.32,77.18 25.94,75.83 25.94,74.13 25.94,73.28 24.69,77.56 27.77,77.18 25.37,72.86 27.17,73.21 27.79,72.83 24.72,73.21
  pour Bottom (no thermals): 17.84,78.66 29.29,78.66 29.29,68.51 20.57,64.91 19.67,67.38 18.82,70.38 18.09,74.56
TH_D63  (via drill 0.35 pad 0.7)
  Top 0.3: D63.TH v70.54,94.83
  Top 0.7: v71.04,91.82 67.96,94.9 v67.69,94.63 70.77,91.56 v71.04,91.82 | v74.11,94.9 71.04,97.97 v70.77,97.71 73.85,94.63 v74.11,94.9
  other vias: 72.34,96.63 69.44,92.92 70.05,93.52 70.65,94.12 71.25,94.72 71.85,95.32 73.17,95.8 72.45,95.92 71.74,96.03 71.65,96.83 71.14,95.43 69.94,94.23 69.34,93.63 71.48,97.53 73.39,95.09 68.63,93.73 70.15,92.71 70.33,92 68.42,94.44
  pour Bottom (no thermals): 72.82,96.72 80.03,89.51 67.02,84.14 60.22,90.94 65.61,103.94 72.84,96.71
TH_D64  (via drill 0.35 pad 0.7)
  Top 0.3: v77.29,79.18 D64.TH
  Top 0.7: v75.52,76.71 75.52,81.06 v75.14,81.06 75.14,76.71 v75.52,76.71 | v79.87,76.71 79.87,81.06 v79.49,81.06 79.49,76.71 v79.87,76.71
  other vias: 79.84,79.18 75.17,78.61 76.02,78.61 76.87,78.61 77.72,78.61 78.57,78.61 79.84,78.01 79.42,78.61 78.99,79.18 79.49,79.81 78.14,79.18 76.44,79.18 75.59,79.18 79.87,80.43 79.49,77.36 75.17,79.76 75.52,77.96 75.14,77.33 75.52,80.41
  pour Bottom (no thermals): 80.17,89.03 80.17,68.63 67.17,74.03 67.17,83.66
TH_D65  (via drill 0.35 pad 0.7)
  Top 0.3: v70.96,63.33 D65.TH
  Top 0.7: v73.86,63.11 70.78,60.04 v71.05,59.77 74.13,62.85 v73.86,63.11 | v70.78,66.19 67.71,63.11 v67.97,62.85 71.05,65.92 v70.78,66.19
  other vias: 69.05,64.42 72.76,61.52 72.16,62.12 71.56,62.72 70.36,63.93 69.88,65.25 69.76,64.53 69.65,63.82 68.86,63.73 70.25,63.22 70.85,62.62 71.46,62.02 72.06,61.42 68.15,63.56 70.59,65.46 71.95,60.71 72.98,62.23 73.68,62.41 71.24,60.5
  pour Bottom (no thermals): 72.83,61.06 65.62,53.84 60.25,66.85 67.05,73.66 80.04,68.27 72.81,61.04
TH_D66  (via drill 0.35 pad 0.7)
  Top 0.3: v55.27,56.61 D66.TH
  Top 0.7: v57.17,54.41 52.82,54.41 v52.82,54.03 57.17,54.03 v57.17,54.41 | v57.17,58.76 52.82,58.76 v52.82,58.38 57.17,58.38 v57.17,58.76
  other vias: 54.69,58.73 55.27,54.06 55.27,54.91 55.27,55.76 55.27,57.46 55.87,58.73 55.27,58.31 54.69,57.88 54.07,58.38 54.69,57.03 54.69,56.18 54.69,55.33 54.69,54.48 53.44,58.76 56.52,58.38 54.12,54.06 55.92,54.41 56.54,54.03 53.47,54.41
  pour Bottom (no thermals): 65.14,53.68 44.74,53.68 50.14,66.68 59.77,66.68
TH_D70  (via drill 0.35 pad 0.7)
  Top 0.3: v38.73,63.03 D70.TH
  Top 0.7: v39.22,60.02 36.15,63.1 v35.88,62.83 38.96,59.76 v39.22,60.02 | v42.3,63.1 39.22,66.17 v38.96,65.91 42.03,62.83 v42.3,63.1
  other vias: 40.53,64.83 37.63,61.12 38.23,61.72 38.83,62.32 39.43,62.92 40.03,63.52 41.36,64 40.64,64.12 39.93,64.23 39.84,65.02 39.33,63.63 38.13,62.43 37.52,61.82 39.66,65.73 41.57,63.29 36.82,61.93 38.34,60.91 38.51,60.2 36.61,62.64
  pour Bottom (no thermals): 37.14,61.04 29.93,68.26 42.94,73.63 49.74,66.83 44.35,53.83 37.12,61.06
TH_D71  (via drill 0.35 pad 0.7)
  Top 0.3: v32.27,79.16 D71.TH
  Top 0.7: v30.49,76.68 30.49,81.03 v30.12,81.03 30.12,76.68 v30.49,76.68 | v34.84,76.68 34.84,81.03 v34.47,81.03 34.47,76.68 v34.84,76.68
  other vias: 34.82,79.16 30.14,78.58 30.99,78.58 31.84,78.58 32.69,78.58 33.54,78.58 34.82,77.98 34.39,78.58 33.97,79.16 34.47,79.78 33.12,79.16 31.42,79.16 30.57,79.16 34.84,80.41 34.47,77.33 30.14,79.73 30.49,77.93 30.12,77.31 30.49,80.38
  pour Bottom (no thermals): 29.79,68.73 29.79,89.13 42.79,83.73 42.79,74.11
TH_D72  (via drill 0.35 pad 0.7)
  Top 0.3: v39.14,95.14 D72.TH
  Top 0.7: v42.04,94.93 38.96,91.85 v39.23,91.59 42.31,94.66 v42.04,94.93 | v38.96,98 35.89,94.93 v36.15,94.66 39.23,97.74 v38.96,98
  other vias: 37.23,96.24 40.94,93.34 40.34,93.94 39.74,94.54 38.54,95.74 38.06,97.07 37.94,96.34 37.83,95.63 37.04,95.55 38.43,95.03 39.04,94.43 39.64,93.83 40.24,93.23 36.33,95.37 38.77,97.28 40.13,92.52 41.16,94.04 41.86,94.22 39.42,92.31
  pour Bottom (no thermals): 37.15,96.71 44.36,103.93 49.74,90.92 42.93,84.11 29.94,89.5 37.17,96.73
TH_D73  (via drill 0.35 pad 0.7)
  Top 0.3: v55.27,101.58 D73.TH
  Top 0.7: v57.17,99.38 52.82,99.38 v52.82,99.01 57.17,99.01 v57.17,99.38 | v57.17,103.73 52.82,103.73 v52.82,103.36 57.17,103.36 v57.17,103.73
  other vias: 54.69,103.71 55.27,99.03 55.27,99.88 55.27,100.73 55.27,102.43 55.87,103.71 55.27,103.28 54.69,102.86 54.07,103.36 54.69,102.01 54.69,101.16 54.69,100.31 54.69,99.46 53.44,103.73 56.52,103.36 54.12,99.03 55.92,99.38 56.54,99.01 53.47,99.38
  pour Bottom (no thermals): 44.84,104.06 65.24,104.06 59.84,91.06 50.22,91.06
USB_DM_FT232
  Top 0.3: IC5.15 88.09,23.89 88.79,23.18 IC1.6
USB_DM_TGTMCU  (via drill 0.35 pad 0.7)
  Top 0.3: U1.6 53.13,20.45 53.54,20.03 53.54,14.93 v52.59,13.98 | v25.54,7.93 25.54,8.98 R1.2
  Bottom 0.3: v25.54,7.93 31.99,1.48 44.24,1.48 48.49,5.73 50.09,5.73 51.59,7.23 51.59,12.98 v52.59,13.98
USB_DP_FT232  (via drill 0.35 pad 0.7)
  Top 0.3: IC5.14 87.64,23.39 v87.99,23.03 | v90.29,23.03 90.7,22.63 IC1.4
  Bottom 0.3: v87.99,23.03 v90.29,23.03
USB_DP_TGTMCU  (via drill 0.35 pad 0.7)
  Top 0.3: U1.5 53.63,20.64 54.09,20.18 54.09,14.33 v53.69,13.93 | v26.34,6.03 26.34,10.5 R2.2
  Bottom 0.3: v53.69,13.93 52.14,12.38 52.14,7.03 50.29,5.18 48.69,5.18 44.44,0.93 31.44,0.93 v26.34,6.03
USBDM_UART_RX  (via drill 0.35 pad 0.7)
  Top 0.3: PROG.7 44.99,25.28 v45.59,24.68 | U1.23 47.09,16.58 v47.49,16.98
  Bottom 0.3: v47.49,16.98 47.49,17.83 47.09,18.23 47.09,23.18 v45.59,24.68
USBDM_UART_TX  (via drill 0.35 pad 0.7)
  Top 0.3: U1.24 44.01,16.07 v43.39,16.68 | PROG.6 37.32,24.01 36.69,23.38 36.69,20.43 37.84,19.28 42.89,19.28 v43.39,18.78
  Bottom 0.3: v43.39,18.78 v43.39,16.68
